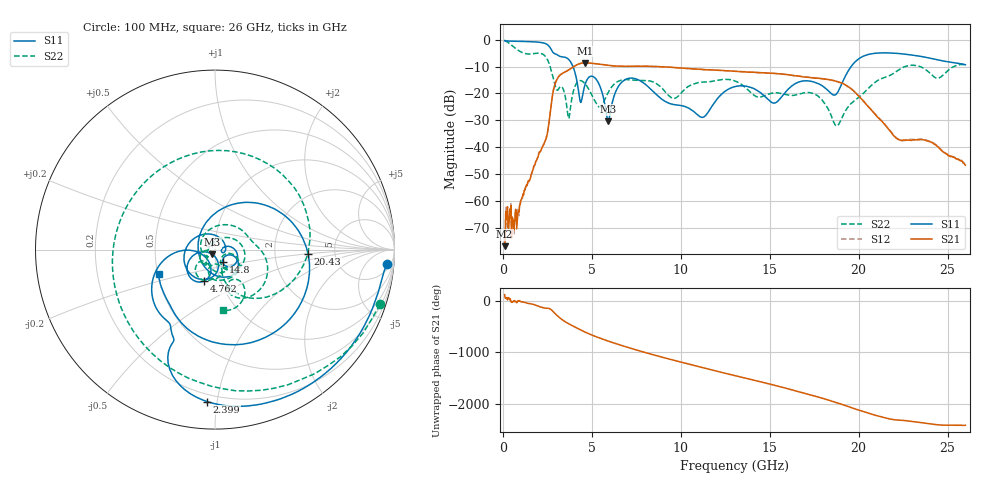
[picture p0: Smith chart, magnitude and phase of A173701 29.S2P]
!  2-Port S-parameters saved by WinCal
! VAR MeasName=S-Parameters (CALIBRATED_DATA) read from VNA (N5245A)
! VAR MeasDate=2017-6-7 10:30:18
! VAR NAME=A173701 29
! VAR FILENAME=A173701 29.S2P
! VAR DATE=2017-6-7 10:30:18
! VAR PHYS_PORTS=1,2
# Hz S DB R 50
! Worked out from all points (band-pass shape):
!   801 points, 100 MHz to 26 GHz, reference 50 ohm
!   highest |S21| = -8.63 dB at 4.633 GHz (marker M1); lowest = -76.9 dB at 100 MHz (marker M2)
!   |S21| within 3 dB of the highest: 3.611 GHz to 12.74 GHz (9.133 GHz wide, 112 % of centre)
!   lowest |S11| = -30.3 dB at 5.928 GHz (marker M3), VSWR 1.06, Z = 48.4 - j2.54 ohm
!   |S11| at or under -10 dB: 3.942 GHz to 19.58 GHz (15.63 GHz wide, 133 % of centre)
!   |S22| runs from -32.1 to -0.3 dB; largest |S21 - S12| = 0.0039
!   S11 on the Smith chart (normalised r, x): 100 MHz: 9, -20; 2.399 GHz: 0.16, -0.94; 4.762 GHz: 0.83, -0.30; 14.8 GHz: 1.08, -0.15; 20.43 GHz: 3.14, -0.19; 26 GHz: 0.51, -0.16
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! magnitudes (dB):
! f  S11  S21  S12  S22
! 100 MHz  -0.3  -76.9  -71.7  -0.3
! 294.2 MHz  -0.5  -70.1  -70.0  -1.0
! 682.8 MHz  -0.6  -66.8  -64.7  -3.0
! 2.399 GHz  -1.4  -37.4  -37.3  -6.3
! 2.949 GHz  -5.3  -16.2  -16.2  -17.4
! 3.694 GHz  -7.3  -11.3  -11.3  -29.4
! 4.438 GHz  -22.3  -8.7  -8.7  -15.4
! 4.633 GHz  -16.5  -8.6  -8.6  -16.5
! 4.762 GHz  -14.6  -8.6  -8.6  -17.7
! 5.41 GHz  -16.6  -9.1  -9.1  -25.0
! 5.928 GHz  -30.3  -9.6  -9.5  -19.6
! 6.963 GHz  -14.6  -9.9  -9.9  -14.8
! 8.744 GHz  -21.1  -10.0  -10.0  -16.9
! 9.618 GHz  -24.2  -10.3  -10.4  -21.9
! 11.24 GHz  -28.9  -11.1  -11.1  -15.8
! 13.05 GHz  -17.5  -11.8  -11.8  -15.4
! 14.8 GHz  -21.6  -12.4  -12.4  -20.6
! 17.39 GHz  -15.6  -14.2  -14.1  -20.0
! 18.78 GHz  -20.0  -15.6  -15.6  -32.1
! 20.43 GHz  -5.7  -24.1  -24.0  -18.9
! 21.69 GHz  -4.9  -33.4  -33.2  -13.5
! 26 GHz  -9.3  -46.7  -46.6  -9.3
